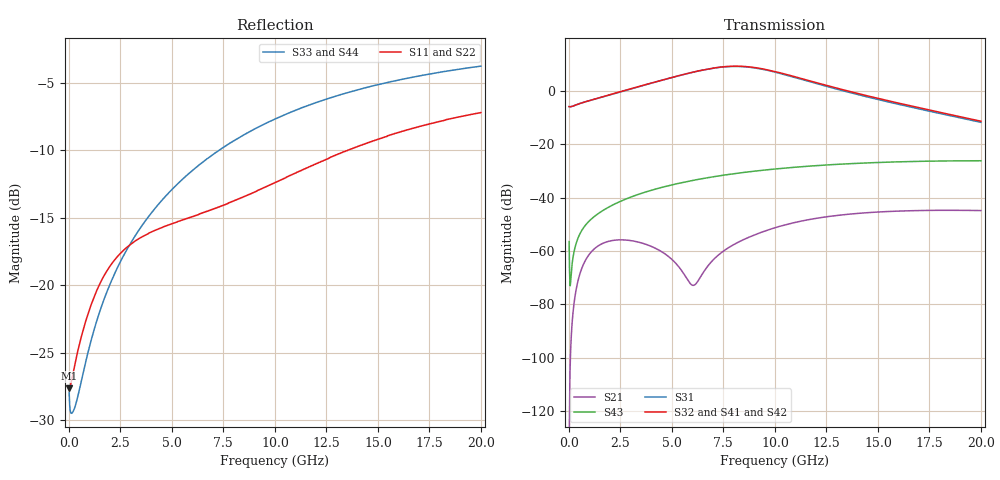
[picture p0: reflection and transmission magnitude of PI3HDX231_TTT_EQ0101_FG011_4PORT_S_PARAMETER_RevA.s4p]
! NPort=4 DATA=2000 NOISE=0 GROUPDELAY=0 COMPLEX_DATAFORMAT=POLAR
! NumOfBlock=1 NumOfParam=0
! .MODEL Smodel S TSTONEFILE=PI3HDX231_TTT_EQ0101_FG011_4PORT_S_PARAMETER_RevA.s4p TYPE=S
!  -- The above .MODEL line can be used for the S element in the netlist.
! The s parameter is extracted from the linear redriver, it is not bi-directional; only s(4,1)s(4,2) and s(3,1)s(3,2)
! should be the insertion loss
!Port definition:
!Port1 = input+
!Port2 = input-
!Port3 = output+
!Port4 = output-
# Hz S MA R  50
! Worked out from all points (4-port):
!   2000 points, 10 MHz to 20 GHz, reference 50 ohm
!   strongest paths, dB at 10 MHz, 5.01 GHz, 10.01 GHz, 15.01 GHz, 20 GHz:
!     S32: -5.9, 5.0, 7.2, -2.9, -11.4
!     S41: -5.9, 5.0, 7.2, -3.0, -11.5
!     S42: -5.9, 5.1, 7.1, -3.1, -11.5
!     S31: -5.9, 5.0, 7.0, -3.3, -11.8
!     S43: -56.5, -35.2, -29.3, -26.9, -26.2
!     S21: -134.8, -63.2, -51.3, -45.4, -44.9
!   lowest |S11| = -27.6 dB at 10 MHz (marker M1), VSWR 1.09, Z = 46 - j0.0776 ohm
!   |S11| at or under -10 dB: start of sweep to 13.55 GHz
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1e7  0.04152 -178.8  1.825e-07 -13.9  0 0.0  0 0.0
     1.825e-07 -14.0  0.04152 -178.8  0 0.0  0 0.0
     0.5042 -0.4  0.5042 179.6  0.04012 -3.2  0.0015 -70.3
     0.5042 179.6  0.5042 -0.4  0.0015 -70.3  0.04012 -3.2
5.17e9  0.1706 -139.8  0.0005954 -13.3  6.947e-10 -174.5  3.524e-10 -150.2
        0.0005982 -13.1  0.1705 -140.0  3.4e-10 -149.8  7.24e-10 -174.6
        1.841 -54.6  1.847 125.0  0.233 -103.0  0.01795 60.7
        1.851 124.8  1.863 -53.6  0.0179 60.6  0.2331 -103.0
7.16e9  0.1932 -135.5  0.000782 100.8  5.361e-09 121.8  2.361e-09 179.6
        0.0007788 99.9  0.1928 -135.7  2.294e-09 -178.9  5.605e-09 120.5
        2.694 -112.4  2.714 67.3  0.311 -108.5  0.02514 48.8
        2.715 66.9  2.734 -111.4  0.02504 48.8  0.3112 -108.5
8.79e9  0.2173 -131.7  0.00186 93.6  1.657e-08 68.2  1.052e-08 137.9
        0.001846 93.1  0.2164 -132.0  1.032e-08 139.6  1.721e-08 66.0
        2.75 -171.3  2.792 8.3  0.3705 -112.7  0.03065 38.4
        2.789 7.9  2.794 -170.2  0.03053 38.5  0.3706 -112.7
1.052e10  0.2496 -129.0  0.003126 78.3  3.709e-08 21.0  3.053e-08 80.9
          0.003104 77.9  0.2482 -129.2  3.018e-08 82.7  3.79e-08 18.3
          1.986 132.9  2.039 -47.8  0.4289 -116.9  0.03586 27.1
          2.032 -48.2  2.02 134.1  0.03574 27.2  0.4289 -116.9
1.316e10  0.3074 -128.2  0.004731 51.0  9.499e-08 -36.9  8.055e-08 5.9
          0.004693 50.7  0.3054 -128.2  8.041e-08 7.7  9.54e-08 -39.5
          1.035 72.6  1.08 -109.2  0.5059 -122.8  0.04231 9.9
          1.072 -109.6  1.057 74.1  0.04222 10.2  0.5059 -122.8
2e10  0.4355 -135.6  0.005758 -4.6  3.766e-07 -160.1  2.779e-07 -134.0
      0.00571 -4.7  0.4338 -135.4  2.803e-07 -133.0  3.705e-07 -162.1
      0.2565 -36.1  0.2691 137.6  0.6464 -135.0  0.04883 -32.3
      0.2654 137.7  0.2668 -34.5  0.04893 -32.0  0.6461 -135.0
